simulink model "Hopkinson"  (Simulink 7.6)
settings: Solver=ode23tb  StartTime=0.0  StopTime=10  RelTol=1e-3
InitFcn:
  | a=1% %0.8;
StopFcn:
  | close all, clc
  | load MMF_flux.mat
  | plotyy(x(1,:),x(2,:),x(1,:),x(3,:))
  | grid
  | title('Flux et reluctance')
  | xlabel('temps')
undefined symbols (not defined in the file or in its folder): sinc
libraries: fl_lib x5, nesl_utility x4

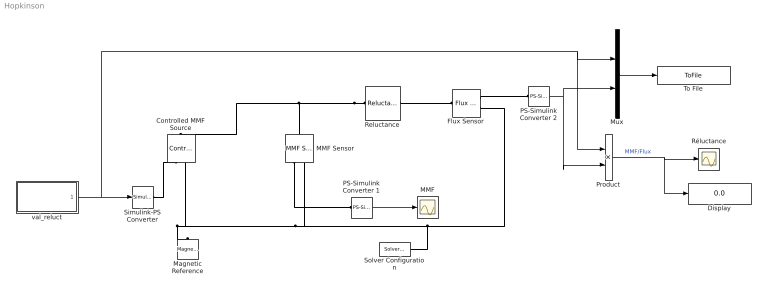
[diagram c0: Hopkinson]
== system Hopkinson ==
  Controlled MMF Source : fl_lib/Magnetic/Magnetic Sources/Controlled MMF Source  DialogController=NetworkEngine.DynNeDlgSource  SystemSampleTime=-1  phi_Log=off  mmf_Log=off  LocalVarNames=|phi|mmf  LocalVarDescs=|phi|mmf  LocalVarLogging=[0 0]
  Display : Display
  Flux Sensor : fl_lib/Magnetic/Magnetic Sensors/Flux Sensor  DialogController=NetworkEngine.DynNeDlgSource  SystemSampleTime=-1  phi_Log=off  mmf_Log=off  LocalVarNames=|phi|mmf  LocalVarDescs=|phi|mmf  LocalVarLogging=[0 0]
  MMF : Scope
  MMF Sensor : fl_lib/Magnetic/Magnetic Sensors/MMF Sensor  DialogController=NetworkEngine.DynNeDlgSource  SystemSampleTime=-1  phi_Log=off  mmf_Log=off  LocalVarNames=|phi|mmf  LocalVarDescs=|phi|mmf  LocalVarLogging=[0 0]
  Magnetic Reference : fl_lib/Magnetic/Magnetic Elements/Magnetic Reference  DialogController=NetworkEngine.DynNeDlgSource  SystemSampleTime=-1  phi_Log=off  LocalVarNames=|phi  LocalVarDescs=|phi  LocalVarLogging=0
  Mux : Mux  Inputs=2
  PS-Simulink Converter 1 : nesl_utility/PS-Simulink Converter  DialogController=NetworkEngine.DynNeUtilDlgSource  SystemSampleTime=-1  PhysicalDomain=network_engine_domain  LeftPortType=input  RightPortType=output  SubClassName=ps_output  Unit=1  AffineConversion=off
  PS-Simulink Converter 2 : nesl_utility/PS-Simulink Converter  DialogController=NetworkEngine.DynNeUtilDlgSource  SystemSampleTime=-1  PhysicalDomain=network_engine_domain  LeftPortType=input  RightPortType=output  SubClassName=ps_output  Unit=1  AffineConversion=off
  Product : Product  Inputs=*/
  Reluctance : fl_lib/Magnetic/Magnetic Elements/Reluctance  DialogController=NetworkEngine.DynNeDlgSource  SystemSampleTime=-1  g=0.3 m  CSA=4e-004 m^2  mur=1  phi_Log=off  mmf_Log=off  LocalVarNames=|phi|mmf  LocalVarDescs=|phi|mmf  LocalVarLogging=[0 0]
  Réluctance : Scope
  Simulink-PS Converter : nesl_utility/Simulink-PS Converter  DialogController=NetworkEngine.DynNeUtilDlgSource  SystemSampleTime=-1  PhysicalDomain=network_engine_domain  LeftPortType=input  RightPortType=output  SubClassName=ps_input  Unit=1  AffineConversion=off  InputFilterTimeConstant=.001  UdotUserProvided=0
  Solver Configuration : nesl_utility/Solver Configuration  DialogController=NetworkEngine.DynNeUtilDlgSource  SystemSampleTime=-1  PhysicalDomain=network_engine_domain  LeftPortType=input  RightPortType=generic  SubClassName=solver  Accelerate=off  Profile=off  ResidualTolerance=1e-9  MaxNonlinIter=3  MaxModeIter=2  DoFixedCost=off  UseLocalSampling=off  DoDC=off  LinearAlgebra=Sparse  LocalSolverSampleTime=.001  LocalSolverChoice=NE_BACKWARD_EULER_ADVANCER  UseLocalSolver=off
  To File : ToFile  Filename=MMF_flux  MatrixName=x
  val_reluct : Subsystem
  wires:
  PS-Simulink Converter 2/1 -> Mux/2, Product/2
  PS-Simulink Converter 1/1 -> MMF/1
  Mux/1 -> To File/1
  val_reluct/1(MMF) -> Simulink-PS Converter/1, Mux/1, Product/1
  Product/1 -> Réluctance/1, Display/1  "MMF/Flux"
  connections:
  Reluctance/LConn1 -- MMF Sensor/LConn1 -- Controlled MMF Source/LConn1
  Flux Sensor/RConn2 -- MMF Sensor/RConn2 -- Controlled MMF Source/RConn2 -- Magnetic Reference/LConn1 -- Solver Configuration/RConn1
  Flux Sensor/RConn1 -- PS-Simulink Converter 2/LConn1
  MMF Sensor/RConn1 -- PS-Simulink Converter 1/LConn1
  Simulink-PS Converter/RConn1 -- Controlled MMF Source/RConn1
  Reluctance/RConn1 -- Flux Sensor/LConn1

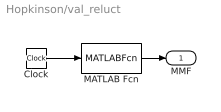
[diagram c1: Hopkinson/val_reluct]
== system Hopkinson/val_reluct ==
  Clock : Clock
  MATLAB Fcn : MATLABFcn  MATLABFcn=sinc(u)+2
  MMF : Outport
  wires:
  Clock/1 -> MATLAB Fcn/1
  MATLAB Fcn/1 -> MMF/1
